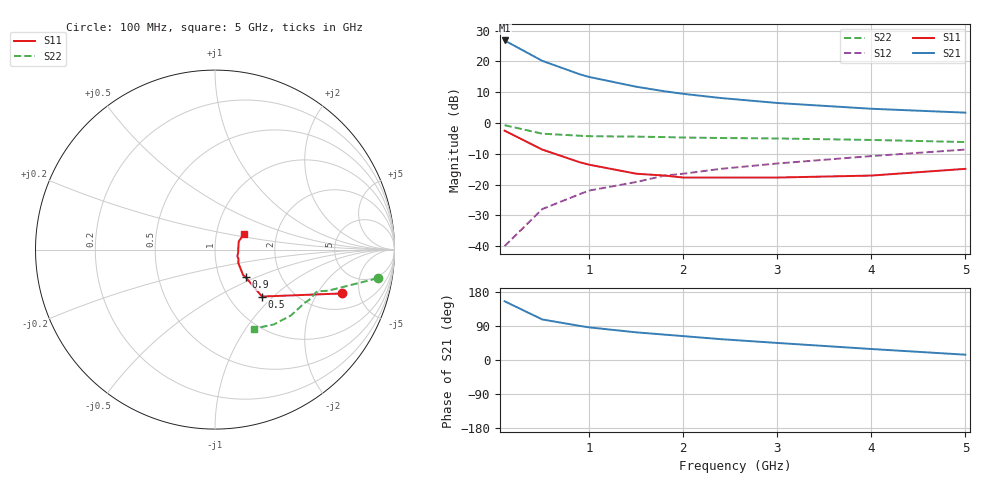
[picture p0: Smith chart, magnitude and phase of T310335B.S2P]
!AT-31033
!S and NOISE PARAMETERS at Vce=5V  Ic=10mA.  LAST UPDATED 04-10-94
# ghz s ma r 50
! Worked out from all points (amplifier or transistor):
!   11 points, 100 MHz to 5 GHz, reference 50 ohm
!   highest |S21| = 26.8 dB at 100 MHz (marker M1)
!   |S21| within 3 dB of that: start of sweep to 281.5 MHz
!   unconditionally stable (mu >= 1): 1.13 GHz to 3.511 GHz
!   at 500 MHz: K = 0.89, MSG = 24.1 dB, |S12| = -28.0 dB
!   at 1.8 GHz: K = 1.01, MAG = 13.1 dB, |S12| = -17.1 dB
!   at 5 GHz: K = 0.94, MSG = 6.0 dB, |S12| = -8.6 dB
!   lowest NFmin = 1.30 dB at 500 MHz
!   S11 on the Smith chart (normalised r, x): 100 MHz: 3.03, -3.39; 500 MHz: 1.41, -0.85; 900 MHz: 1.33, -0.43; 5 GHz: 1.35, +0.24
0.1  0.75 -19.0  21.84 155.0  0.01 79.0  0.92 -10.0
0.5  0.37 -45.0  10.2 107.0  0.04 73.0  0.67 -20.0
0.9  0.23 -42.0  6.16 90.0  0.07 72.0  0.62 -22.0
1  0.21 -42.0  5.58 86.0  0.08 72.0  0.61 -23.0
1.5  0.15 -30.0  3.87 73.0  0.11 69.0  0.6 -27.0
1.8  0.14 -21.0  3.27 67.0  0.14 66.0  0.59 -29.0
2  0.13 -17.0  2.97 63.0  0.15 65.0  0.58 -31.0
2.4  0.13 -7.0  2.54 55.0  0.18 62.0  0.57 -35.0
3  0.13 3.0  2.11 45.0  0.22 57.0  0.56 -41.0
4  0.14 19.0  1.7 29.0  0.29 48.0  0.53 -52.0
5  0.18 28.0  1.47 14.0  0.37 38.0  0.49 -64.0
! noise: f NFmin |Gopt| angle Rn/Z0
0.5  1.3  0.42  10  0.38
0.9  1.4  0.31  30  0.34
1.8  1.7  0.16  80  0.23
2.4  2  0.08  118  0.17
